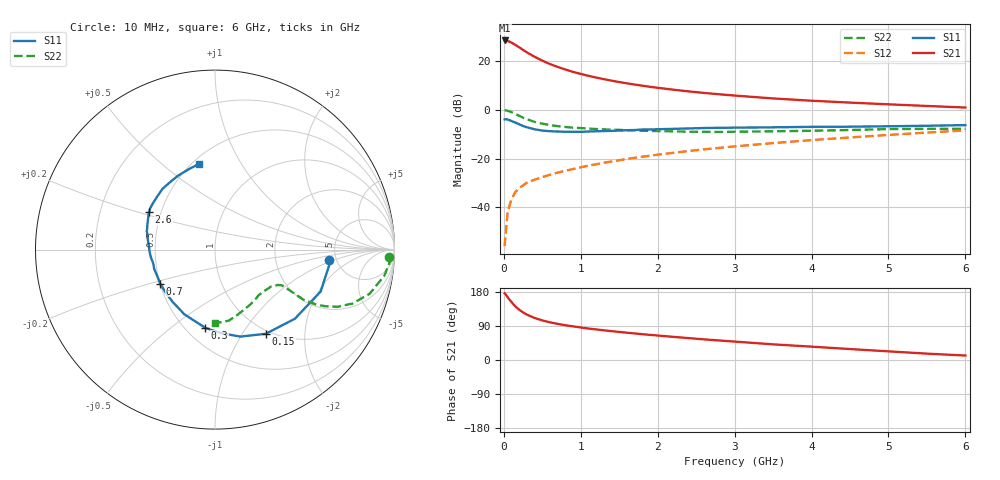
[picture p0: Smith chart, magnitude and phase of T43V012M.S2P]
! Infineon Technologies  Discrete & RF Semiconductors
! BFR182T
! Si NPN RF Bipolar Junction Transistor in SC75
! VCE = 3 V  IC = 12 mA
! Common Emitter S-Parameters:  October  1999
# GHz  S  MA  R  50
!  f  S11  S21  S12  S22
! GHz  MAG  ANG  MAG  ANG  MAG  ANG  MAG  ANG
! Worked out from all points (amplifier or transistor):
!   36 points, 10 MHz to 6 GHz, reference 50 ohm
!   highest |S21| = 28.4 dB at 10 MHz (marker M1)
!   |S21| within 3 dB of that: start of sweep to 208.5 MHz
!   unconditionally stable (mu >= 1): 878.3 MHz to 3.744 GHz
!   at 250 MHz: K = 0.51, MSG = 27.8 dB, |S12| = -31.0 dB
!   at 1.4 GHz: K = 1.09, MAG = 14.8 dB, |S12| = -21.2 dB
!   at 6 GHz: K = 0.84, MSG = 4.7 dB, |S12| = -8.5 dB
!   S11 on the Smith chart (normalised r, x): 10 MHz: 4.32, -0.85; 150 MHz: 0.95, -1.28; 300 MHz: 0.62, -0.67; 700 MHz: 0.50, -0.22; 2.6 GHz: 0.43, +0.22; 6 GHz: 0.54, +0.67
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0.01  0.636 -5.3  26.44 176.0  0.0016 85.2  0.9695 -2.4
0.02  0.6428 -7.4  26.32 174.2  0.0025 86.2  0.9794 -3.5
0.05  0.6334 -21.6  25.86 165.4  0.0081 79.9  0.9549 -8.7
0.1  0.5886 -40.9  23.84 152.7  0.0147 76.2  0.8956 -16.0
0.15  0.5477 -58.9  21.48 141.4  0.0206 67.5  0.8217 -21.5
0.2  0.5047 -73.8  19.11 132.6  0.0248 66.0  0.7535 -25.0
0.25  0.4662 -86.0  16.92 125.6  0.0282 61.3  0.6901 -27.2
0.3  0.4394 -97.1  15.06 119.7  0.032 60.8  0.6418 -28.5
0.4  0.3987 -115.4  12.23 110.8  0.0369 59.1  0.5658 -29.5
0.5  0.3753 -128.7  10.19 104.5  0.0417 60.5  0.5196 -29.1
0.6  0.3641 -139.6  8.675 99.4  0.0466 61.1  0.4865 -28.8
0.7  0.3593 -148.2  7.571 95.3  0.0515 62.6  0.4622 -28.5
0.9  0.3557 -162.3  5.996 88.7  0.0611 64.3  0.4302 -28.2
1.1  0.3592 -172.9  4.977 83.0  0.0719 65.8  0.4125 -28.7
1.3  0.3669 179.2  4.257 78.3  0.0823 66.7  0.3974 -29.9
1.6  0.3822 169.6  3.489 72.0  0.0984 67.5  0.3815 -32.0
2.2  0.4068 157.0  2.589 61.1  0.1312 67.7  0.3618 -38.6
2.6  0.4233 150.4  2.223 54.5  0.1545 67.1  0.3537 -43.8
3.5  0.4376 137.2  1.712 41.3  0.2076 64.2  0.3628 -56.5
4.5  0.4508 124.4  1.406 28.9  0.2712 59.6  0.3856 -71.6
5.5  0.4708 108.3  1.199 16.8  0.3417 53.8  0.407 -84.7
6  0.4857 100.6  1.114 11.8  0.378 50.1  0.4066 -90.0
